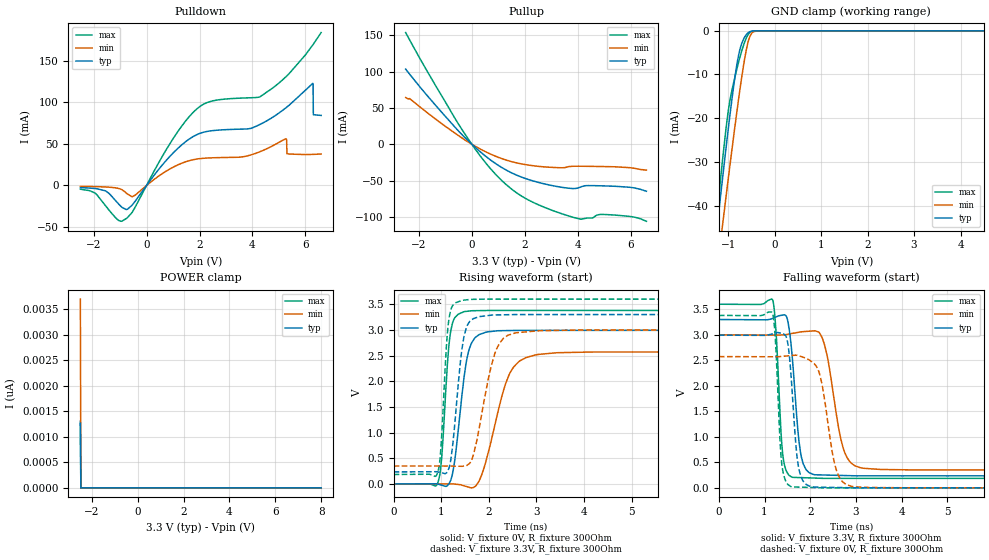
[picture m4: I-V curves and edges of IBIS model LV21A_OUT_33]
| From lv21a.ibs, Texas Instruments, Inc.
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|   Model LV21A_OUT_33
[Model]   LV21A_OUT_33
Model_type   Output
Polarity   Non-Inverting
Vmeas = 1.65
Vref = 0
Cref = 2pF
Rref = 100000
|   typ   min   max
C_comp   5.7pF   5.6pF   6pF
[Voltage Range]   3.3   3   3.6
[Temperature Range]   25   125   -40
[Pullup Reference]   3.3   3   3.6
[Pulldown Reference]   0   0   0
[Power Clamp Reference]   3.3   3   3.6
[GND Clamp Reference]   0   0   0
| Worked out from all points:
|   slope of the pulldown table from 0 to 0.495 V, typ, clamps not added: 23.8 ohm
|   slope of the pullup table from 0 to 0.495 V, typ, clamps not added: 31.6 ohm
|   GND clamp passes 1 mA (typ) near -0.62 V on its own axis
|   falling waveform, V_fixture 3.3V, R_fixture 300Ohm: 20-80 % time 170ps typ, 296ps min, 115ps max; typ from 3.3 V to 0.235 V
|   rising waveform, V_fixture 0V, R_fixture 300Ohm: 20-80 % time 227ps typ, 437ps min, 140ps max; typ from 0 V to 2.99 V
|   rising waveform, V_fixture 3.3V, R_fixture 300Ohm: 20-80 % time 194ps typ, 349ps min, 123ps max; typ from 0.235 V to 3.3 V
|   falling waveform, V_fixture 0V, R_fixture 300Ohm: 20-80 % time 151ps typ, 272ps min, 106ps max; typ from 2.99 V to 0 V
[Pulldown]
|   Voltage   I(typ)   I(min)   I(max)
-2.5V     -2.551mA   -1.061mA   -4.505mA
-1.555V   -6.484mA   -1.819mA   -24.18mA
-767.5mV  -29mA      -9.023mA   -39.85mA
1.805V    59.64mA    31.28mA    89.38mA
4.272V    73.26mA    40.48mA    106.5mA
5.26V     93.35mA    56.14mA    130.7mA
5.291V    94.15mA    54.17mA    131.7mA
5.301V    94.42mA    38.19mA    132mA
6.278V    122.9mA    37.37mA    169.1mA
6.288V    121.8mA    37.38mA    169.6mA
6.299V    85.16mA    37.39mA    170mA
6.593V    84.29mA    37.83mA    184mA
[GND Clamp]
|   Voltage   I(typ)   I(min)   I(max)
-2.5V     -170.7mA   -168.9mA   -187.4mA
-1.282V   -49.09mA   -58.54mA   -46.61mA
-1.24V    -45.04mA   -54.83mA   -42.02mA
-1.208V   -42.02mA   -52.06mA   -38.61mA
-1.125V   -34.05mA   -44.71mA   -29.82mA
-977.5mV  -20.62mA   -32.07mA   -16.86mA
-799mV    -6.847mA   -17.4mA    -8.124mA
-715mV    -3.091mA   -11.05mA   -4.817mA
-641.5mV  -1.357mA   -6.134mA   -2.454mA
-526mV    -161.3uA   -1.092mA   -287.1uA
-379mV    -1.458uA   -24.15uA   -787.7nA
8V        0A         0A         0A
[Pullup]
|   Voltage   I(typ)   I(min)   I(max)
-2.5V     103.5mA    64.33mA    153.8mA
-2.353V   96.65mA    63mA       143.9mA
-620.5mV  22.91mA    14.86mA    34.6mA
-11.5mV   394.6uA    251uA      611.5uA
723.5mV   -22.08mA   -13.78mA   -34.35mA
1.5V      -39.33mA   -23.88mA   -61.67mA
2.487V    -52.23mA   -30.27mA   -82.86mA
3.958V    -60.61mA   -30.21mA   -101.8mA
4.545V    -56.9mA    -30.43mA   -101.5mA
4.987V    -57.31mA   -30.68mA   -96.63mA
6.099V    -59.86mA   -32.84mA   -100mA
6.593V    -64.68mA   -35.58mA   -106mA
[POWER Clamp]
|   Voltage   I(typ)   I(min)   I(max)
-2.5V     1.265nA    3.699nA    1.306nA
-2.479V   0A         0A         0A
-2.469V   0A         0A         0A
8V        0A         0A         0A
[Ramp]
R_load = 300
|   typ   min   max
dV/dt_r   1.7962/2.27118e-10   1.54366/4.32572e-10   2.0282/1.3953e-10
dV/dt_f   1.83881/1.68896e-10   1.58975/2.95162e-10   2.04844/1.15376e-10
[Falling Waveform]
V_fixture = 3.3V
V_fixture_min = 3V
V_fixture_max = 3.6V
R_fixture = 300Ohm
C_fixture = 0F
|   Time   V(typ)   V(min)   V(max)
0s        3.3V       3V         3.6V
1.178ns   3.323V     2.995V     3.68V
1.394ns   3.386V     2.999V     689.7mV
1.6ns     2.631V     3.027V     209.4mV
1.756ns   897.8mV    3.051V     201.9mV
1.901ns   369.6mV    3.066V     197.6mV
2.268ns   252.7mV    2.926V     186.8mV
2.72ns    242.6mV    786.6mV    186.2mV
3.096ns   235.8mV    396mV      186.2mV
15ns      235.3mV    350.4mV    185.9mV
[Rising Waveform]
V_fixture = 0V
V_fixture_min = 0V
V_fixture_max = 0V
R_fixture = 300Ohm
C_fixture = 0F
|   Time   V(typ)   V(min)   V(max)
0s        6.111uV    3.164uV    7.427uV
925.7ps   -88.09uV   2.381mV    16.97mV
1.009ns   -22.89mV   2.596mV    508.6mV
1.192ns   57.45mV    3.066mV    2.933V
1.474ns   2.034V     -33.27mV   3.354V
1.59ns    2.63V      -65.28mV   3.368V
1.798ns   2.91V      63.03mV    3.376V
2.425ns   2.988V     2.124V     3.379V
2.978ns   2.992V     2.513V     3.379V
15ns      2.994V     2.573V     3.38V
[Rising Waveform]
V_fixture = 3.3V
V_fixture_min = 3V
V_fixture_max = 3.6V
R_fixture = 300Ohm
C_fixture = 0F
|   Time   V(typ)   V(min)   V(max)
0s        235.3mV    350.4mV    185.9mV
917.4ps   235.9mV    351.2mV    198.9mV
989.5ps   223.8mV    351.2mV    655.7mV
1.105ns   213.4mV    349.8mV    2.63V
1.16ns    303.3mV    349mV      3.197V
1.431ns   2.594V     345.2mV    3.573V
1.673ns   3.219V     558mV      3.596V
2.145ns   3.292V     2.589V     3.6V
2.56ns    3.299V     2.942V     3.6V
15ns      3.3V       3V         3.6V
[Falling Waveform]
|Gnd
V_fixture = 0V
V_fixture_min = 0V
V_fixture_max = 0V
R_fixture = 300Ohm
C_fixture = 0F
|   Time   V(typ)   V(min)   V(max)
0s        2.994V     2.573V     3.38V
1.173ns   3.019V     2.57V      3.428V
1.375ns   3.028V     2.577V     479.1mV
1.579ns   2.203V     2.593V     22.66mV
1.707ns   648.4mV    2.599V     15.69mV
1.834ns   149.2mV    2.564V     12.32mV
2.183ns   14.82mV    2.294V     3.065mV
2.56ns    7.702mV    386.4mV    255.5uV
2.9ns     1.284mV    30.14mV    248.7uV
15ns      6.585uV    4.405uV    7.531uV
